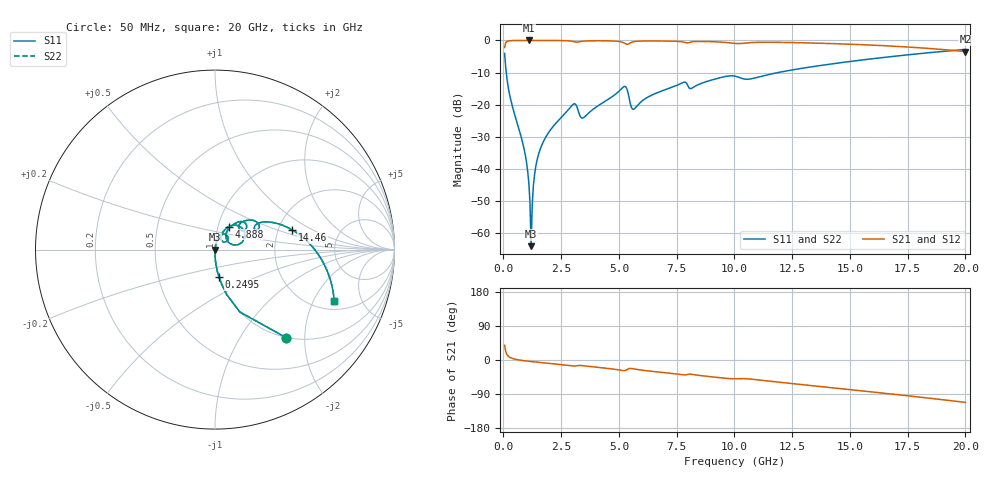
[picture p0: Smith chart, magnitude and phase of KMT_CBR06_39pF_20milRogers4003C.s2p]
! Data measured by Modelithics Inc. support@modelithics.com 813-866-6335
! KEMET CBR0603 39pF, Pad Width= 0.851mm, Pad Length= 0.64mm, Pad Gap= 0.62mm, 20mil Rogers 4003C substrate Data, January 2022
# hz S ma R 50
! 2 Port Network Data from SP1.SP block
! freq  magS11  angS11  magS21  angS21  magS12  angS12  magS22  angS22
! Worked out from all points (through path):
!   401 points, 50 MHz to 20 GHz, reference 50 ohm
!   highest |S21| = -0.01 dB at 1.097 GHz (marker M1); lowest = -3.5 dB at 20 GHz (marker M2)
!   group delay of S21, straight-line fit = 15.6 ps
!   lowest |S11| = -64.1 dB at 1.197 GHz (marker M3), VSWR 1.00, Z = 50.1 - j0.0127 ohm
!   |S11| at or under -10 dB: 122.4 MHz to 11.89 GHz (11.77 GHz wide, 196 % of centre)
!   |S22| runs from -64.1 to -2.8 dB; largest |S21 - S12| = 0
!   S11 on the Smith chart (normalised r, x): 50 MHz: 1.00, -1.62; 249.5 MHz: 1.00, -0.31; 4.888 GHz: 1.12, +0.29; 14.46 GHz: 2.38, +0.65; 20 GHz: 2.45, -2.94
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5e7  0.6295 -51.1  0.7765 38.8  0.7765 38.8  0.6295 -51.1
2.495e8  0.1539 -81.8  0.9876 8.0  0.9876 8.0  0.1539 -81.8
8.97875e8  0.02006 -90.4  0.9992 -1.9  0.9992 -1.9  0.02006 -90.4
1.0475e9  0.00931 -89.5  0.9993 -3.1  0.9993 -3.1  0.00931 -89.5
1.097375e9  0.006112 -87.9  0.9994 -3.4  0.9994 -3.4  0.006112 -87.9
1.197125e9  0.0006261 -11.7  0.9993 -4.1  0.9993 -4.1  0.0006261 -11.7
1.296875e9  0.005515 78.5  0.9993 -4.8  0.9993 -4.8  0.005515 78.5
1.34675e9  0.008153 80.2  0.9992 -5.1  0.9992 -5.1  0.008153 80.2
1.4465e9  0.01324 81.2  0.9992 -5.7  0.9992 -5.7  0.01324 81.2
1.8455e9  0.03193 80.2  0.9985 -8.1  0.9985 -8.1  0.03193 80.2
2.992625e9  0.09947 59.7  0.9703 -15.8  0.9703 -15.8  0.09947 59.7
3.391625e9  0.06174 47.3  0.9694 -14.7  0.9694 -14.7  0.06174 47.3
4.887875e9  0.1489 59.1  0.9739 -25.2  0.9739 -25.2  0.1489 59.1
5.286875e9  0.1912 30.6  0.8851 -27.3  0.8851 -27.3  0.1912 30.6
5.636e9  0.08467 37.2  0.9556 -23.4  0.9556 -23.4  0.08467 37.2
6.73325e9  0.1571 55.5  0.9802 -31.9  0.9802 -31.9  0.1571 55.5
1.0025e10  0.2778 27.3  0.899 -49.5  0.899 -49.5  0.2778 27.3
1.067338e10  0.251 29.3  0.9229 -50.2  0.9229 -50.2  0.251 29.3
1.336662e10  0.3897 21.1  0.9112 -67.6  0.9112 -67.6  0.3897 21.1
1.446388e10  0.4433 14.4  0.8871 -74.5  0.8871 -74.5  0.4433 14.4
1.670825e10  0.5563 -0.1  0.8202 -89.0  0.8202 -89.0  0.5563 -0.1
2e10  0.7235 -23.3  0.6702 -111.8  0.6702 -111.8  0.7235 -23.3
